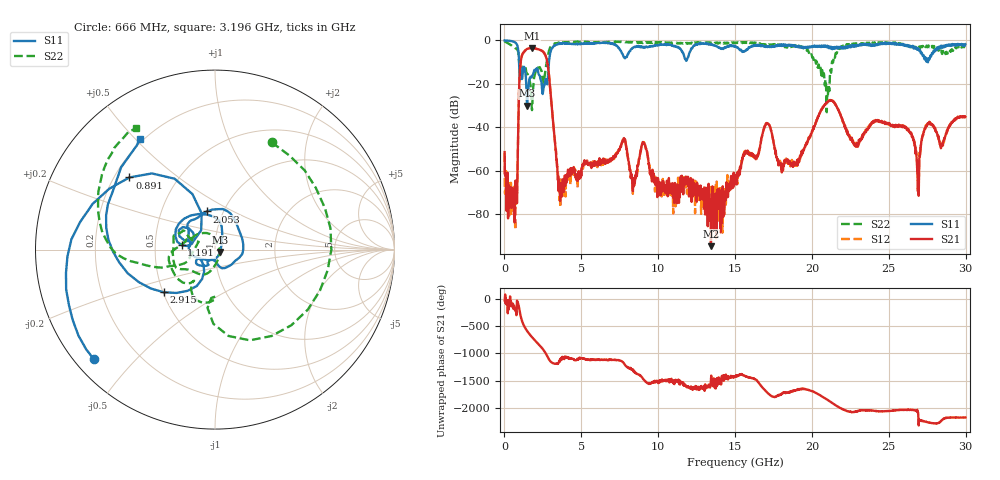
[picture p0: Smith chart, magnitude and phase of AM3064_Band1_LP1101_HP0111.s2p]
# Hz S DB R 50.0
!freq dBS11 angS11 dBS21 angS21 dBS12 angS12 dBS22 angS22
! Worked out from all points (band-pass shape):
!   1600 points, 10 MHz to 29.98 GHz, reference 50 ohm
!   highest |S21| = -3.47 dB at 1.791 GHz (marker M1); lowest = -94.6 dB at 13.43 GHz (marker M2)
!   |S21| within 3 dB of the highest: 1.164 GHz to 2.641 GHz (1.477 GHz wide, 77.6 % of centre)
!   lowest |S11| = -30.1 dB at 1.472 GHz (marker M3), VSWR 1.06, Z = 52.9 - j1.35 ohm
!   |S11| at or under -10 dB: 949.6 MHz to 2.894 GHz (1.945 GHz wide, 101 % of centre); 27.53695 GHz to 27.54645 GHz (9.499 MHz wide, 0.0345 % of centre)
!   |S22| runs from -33.0 to -0.4 dB; largest |S21 - S12| = 0.01
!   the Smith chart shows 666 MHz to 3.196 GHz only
!   S11 on the Smith chart (normalised r, x): 666 MHz: 0.05, -0.38; 891 MHz: 0.26, +0.34; 1.191 GHz: 0.69, +0.03; 2.053 GHz: 0.84, +0.37; 2.915 GHz: 0.50, -0.28; 3.196 GHz: 0.19, +0.52
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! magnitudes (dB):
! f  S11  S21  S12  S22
! 10 MHz  0.0  -51.3  -51.8  -0.4
! 666 MHz  -0.8  -83.7  -66.9  -3.4
! 891 MHz  -4.1  -42.5  -42.6  -5.3
! 1.191 GHz  -14.5  -6.0  -6.0  -12.7
! 1.472 GHz  -30.1  -3.9  -3.9  -15.4
! 1.791 GHz  -16.5  -3.5  -3.5  -32.1
! 2.053 GHz  -13.2  -3.9  -3.8  -13.1
! 2.915 GHz  -8.6  -17.4  -17.4  -4.3
! 3.196 GHz  -2.5  -40.2  -39.8  -1.9
! 3.628 GHz  -1.4  -73.8  -76.8  -1.1
! 5.015 GHz  -1.6  -59.5  -58.9  -0.7
! 9.063 GHz  -3.0  -47.4  -47.3  -1.1
! 10 GHz  -2.1  -64.6  -64.4  -0.9
! 13.43 GHz  -2.0  -94.6  -67.4  -1.3
! 15 GHz  -2.9  -63.8  -62.5  -1.3
! 17.05 GHz  -2.9  -38.2  -37.9  -2.3
! 18.02 GHz  -1.8  -57.6  -56.6  -2.5
! 19.99 GHz  -3.1  -42.2  -42.2  -7.0
! 20.98 GHz  -2.6  -28.5  -28.2  -26.2
! 25 GHz  -1.1  -38.3  -37.9  -1.2
! 26.89 GHz  -3.9  -69.3  -64.8  -3.3
! 29.98 GHz  -1.8  -35.1  -35.2  -2.9
